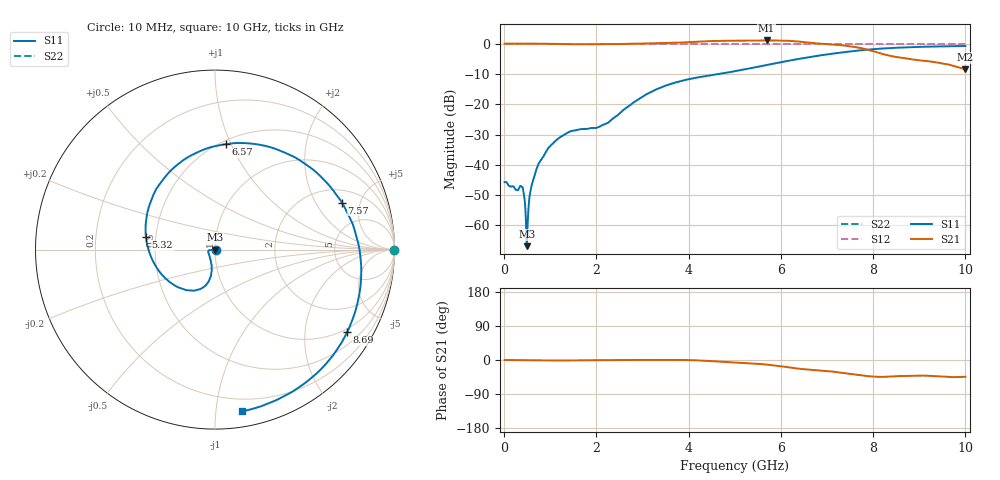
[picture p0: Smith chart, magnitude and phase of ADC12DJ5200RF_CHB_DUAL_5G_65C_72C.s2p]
! Texas Instruments, Inc.
! ADC12DJ5200RF - CH B S-Parameters (Dual Ch Mode, Fs = 5 GSPS, 65 degC case, 72 degC juntion)
! Port 1 represents the 100-ohm differenal input, Port 2 the digital output
! freq  dbS11  angS11  dbS21 angS21 dbS12 angS12 dbS22 angS22
# HZ S DB R 100
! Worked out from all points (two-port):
!   1000 points, 10 MHz to 10 GHz, reference 100 ohm
!   highest |S21| = 1.06 dB at 5.69 GHz (marker M1); lowest = -8.4 dB at 10 GHz (marker M2)
!   |S21| within 3 dB of the highest: start of sweep to 7.864 GHz
!   lowest |S11| = -66.8 dB at 490 MHz (marker M3), VSWR 1.00, Z = 100 + j0.0909 ohm
!   |S11| at or under -10 dB: start of sweep to 4.655 GHz
!   |S22| runs from 0.0 to 0.0 dB; largest |S21 - S12| = 0.77
!   S11 on the Smith chart (normalised r, x): 10 MHz: 1.01, -0.00; 5.32 GHz: 0.44, +0.07; 6.57 GHz: 0.53, +0.96; 7.57 GHz: 2.79, +3.39; 8.69 GHz: 0.87, -3.26; 10 GHz: 0.11, -1.18
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1e7  -45.69 -2.8  0.00 -0.0  0.00 0.0  0.00 0.0
3.8e8  -47.17 -16.4  0.01 -0.5  0.00 0.0  0.00 0.0
4.9e8  -66.84 93.5  0.00 -0.6  0.00 0.0  0.00 0.0
5.2e8  -56.15 -177.4  0.00 -0.7  0.00 0.0  0.00 0.0
5.8e8  -47.93 -158.5  0.00 -0.7  0.00 0.0  0.00 0.0
6.5e8  -44.16 -162.0  -0.02 -0.8  0.00 0.0  0.00 0.0
9.2e8  -35.36 -172.3  -0.02 -1.0  0.00 0.0  0.00 0.0
1.25e9  -30.53 -174.5  -0.12 -1.3  0.00 0.0  0.00 0.0
1.68e9  -28.19 -167.0  -0.20 -0.8  0.00 0.0  0.00 0.0
2.22e9  -26.31 -127.8  -0.14 -0.5  0.00 0.0  0.00 0.0
3.34e9  -14.84 -101.2  0.14 0.1  0.00 0.0  0.00 0.0
4.23e9  -11.08 -126.9  0.69 -1.2  0.00 0.0  0.00 0.0
5.01e9  -9.07 -169.7  0.94 -6.7  0.00 0.0  0.00 0.0
5.32e9  -8.17 169.9  0.95 -8.6  0.00 0.0  0.00 0.0
5.69e9  -7.06 144.7  1.06 -12.2  0.00 0.0  0.00 0.0
6.57e9  -4.57 84.1  0.42 -25.0  0.00 0.0  0.00 0.0
6.67e9  -4.31 77.3  0.25 -26.2  0.00 0.0  0.00 0.0
7.09e9  -3.36 49.3  -0.24 -30.1  0.00 0.0  0.00 0.0
7.57e9  -2.45 20.4  -1.03 -37.7  0.00 0.0  0.00 0.0
8.34e9  -1.48 -18.1  -3.91 -44.0  0.00 0.0  0.00 0.0
8.69e9  -1.23 -32.1  -4.81 -42.4  0.00 0.0  0.00 0.0
1e10  -0.78 -80.5  -8.45 -44.1  0.00 0.0  0.00 0.0
